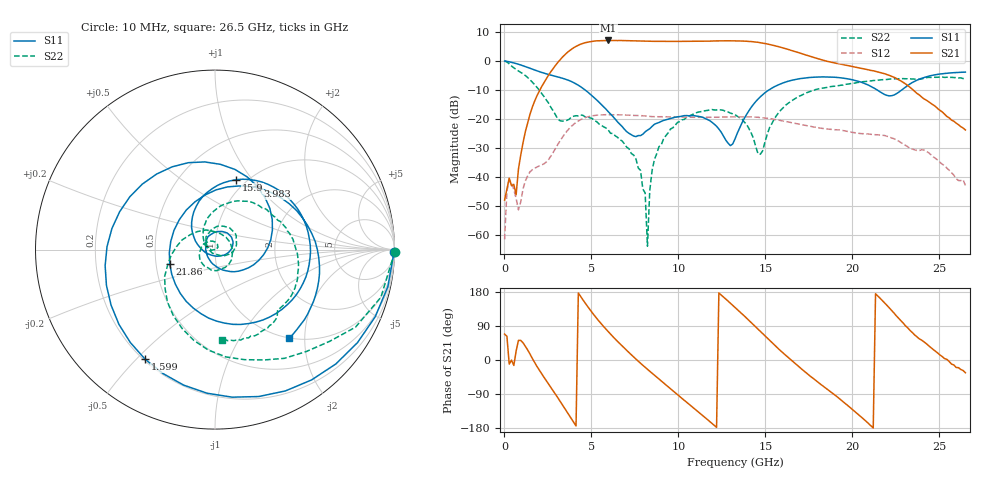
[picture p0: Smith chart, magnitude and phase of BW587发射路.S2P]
!Agilent Technologies,N5242A,MY52422126,A.09.90.01
!Agilent N5242A: A.09.90.01
!Date: Thursday, November 19, 2015 18:56:55
!Correction: S11(Full 2 Port(1,2))
!S21(Full 2 Port(1,2))
!S12(Full 2 Port(1,2))
!S22(Full 2 Port(1,2))
!S2P File: Measurements: S11, S21, S12, S22:
# Hz S  dB  R 50
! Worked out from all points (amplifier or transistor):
!   201 points, 10 MHz to 26.5 GHz, reference 50 ohm
!   highest |S21| = 7.1 dB at 5.97 GHz (marker M1)
!   |S21| within 3 dB of that: 3.86 GHz to 16.27 GHz (12.41 GHz wide, 123 % of centre)
!   unconditionally stable (mu >= 1): 14.1 MHz to end of sweep
!   at 4.381 GHz: K = 2.37, MAG = 6.4 dB, |S12| = -20.2 dB
!   at 13.26 GHz: K = 2.14, MAG = 7.0 dB, |S12| = -19.2 dB
!   at 26.5 GHz: K = 465.57, MAG = -20.1 dB, |S12| = -42.8 dB
!   S11 on the Smith chart (normalised r, x): 10 MHz: open; 1.599 GHz: 0.21, -0.53; 3.983 GHz: 1.16, +0.99; 15.9 GHz: 0.90, +0.84; 21.86 GHz: 0.59, -0.10; 26.5 GHz: 0.99, -1.67
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1e7  -0.02 -0.9  -47.89 68.4  -61.43 66.2  0.01 -0.8
2.749e8  -0.28 -22.8  -40.32 -10.8  -40.90 11.4  -0.97 -28.9
6.7225e8  -0.88 -53.5  -46.07 23.6  -47.33 -77.3  -2.87 -57.4
1.5994e9  -2.80 -122.5  -15.95 4.5  -37.46 80.5  -7.25 -122.5
2.79145e9  -5.06 148.2  -2.67 -80.6  -31.59 69.7  -17.06 134.2
3.9835e9  -7.46 56.3  4.58 -164.5  -21.79 22.8  -18.99 -46.7
4.5133e9  -9.43 18.8  6.05 158.7  -19.78 -6.5  -18.73 -100.9
5.97025e9  -17.46 -62.0  7.07 74.5  -18.50 -73.9  -23.76 143.2
7.82455e9  -25.69 171.1  6.88 -8.6  -18.80 -137.3  -37.66 29.9
8.2219e9  -23.80 144.1  6.80 -24.5  -19.01 -149.4  -63.75 -151.5
8.4868e9  -22.53 127.0  6.76 -34.8  -19.15 -156.7  -37.74 -169.8
8.88415e9  -21.18 104.6  6.77 -50.2  -19.20 -167.2  -29.51 177.8
1.073845e10  -18.81 41.8  6.79 -121.4  -19.38 141.6  -18.60 95.6
1.206295e10  -21.75 -6.8  6.90 -172.5  -19.37 105.8  -16.86 50.2
1.3255e10  -26.85 -147.9  6.93 138.9  -19.24 71.1  -18.50 8.1
1.444705e10  -13.98 130.6  6.52 87.2  -19.34 33.4  -29.45 -61.0
1.5904e10  -7.81 73.1  4.69 23.2  -20.54 -14.3  -16.79 115.0
1.77583e10  -5.59 14.2  1.26 -48.8  -22.70 -68.3  -10.19 60.7
2.01424e10  -6.67 -60.5  -2.08 -136.1  -24.69 -138.5  -7.62 14.6
2.186425e10  -11.56 -162.5  -4.40 150.3  -25.66 162.6  -6.41 -14.6
2.212915e10  -12.01 169.6  -4.94 137.3  -26.15 150.7  -6.24 -19.3
2.65e10  -3.83 -50.3  -23.74 -33.7  -42.83 0.7  -5.94 -85.5
